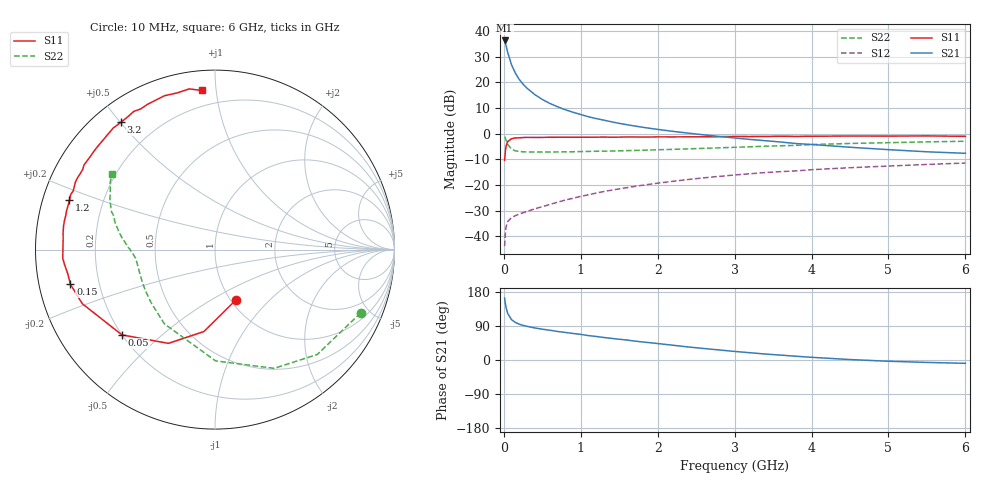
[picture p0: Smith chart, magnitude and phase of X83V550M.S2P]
! SIEMENS Small Signal Semiconductors
! BFP136W
! Si NPN RF Bipolar Junction Transistor in SOT343
! VCE = 3.5 V  IC = 50 mA
! Common Emitter S-Parameters:  September  1994
# GHz  S  MA  R  50
!  f  S11  S21  S12  S22
! GHz  MAG  ANG  MAG  ANG  MAG  ANG  MAG  ANG
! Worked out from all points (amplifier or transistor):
!   40 points, 10 MHz to 6 GHz, reference 50 ohm
!   highest |S21| = 36.4 dB at 10 MHz (marker M1)
!   |S21| within 3 dB of that: start of sweep to 36.94 MHz
!   unconditionally stable (mu >= 1): 683.3 MHz to 2.866 GHz
!   at 200 MHz: K = 0.54, MSG = 26.3 dB, |S12| = -31.3 dB
!   at 1.5 GHz: K = 1.11, MAG = 10.7 dB, |S12| = -21.5 dB
!   at 6 GHz: K = 0.96, MSG = 1.9 dB, |S12| = -11.4 dB
!   S11 on the Smith chart (normalised r, x): 10 MHz: 1.06, -0.65; 50 MHz: 0.20, -0.38; 150 MHz: 0.10, -0.12; 1.2 GHz: 0.08, +0.16; 3.2 GHz: 0.08, +0.50; 6 GHz: 0.11, +0.92
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0.01  0.3032 -67.2  66.02 163.4  0.0064 72.9  0.8846 -23.5
0.02  0.4607 -97.7  58.85 148.9  0.0115 62.2  0.8163 -45.7
0.03  0.5833 -116.4  51.7 137.7  0.0154 53.3  0.7392 -63.5
0.05  0.7033 -137.5  38.64 122.9  0.0193 40.0  0.62 -89.7
0.1  0.7983 -157.8  22.14 106.5  0.0231 32.6  0.5007 -124.3
0.15  0.8285 -166.5  15.21 99.1  0.0253 33.6  0.4627 -140.4
0.2  0.8319 -171.0  11.47 94.6  0.0271 33.8  0.4498 -149.5
0.25  0.8432 -174.5  9.261 91.4  0.0287 36.2  0.4442 -155.3
0.3  0.8494 -176.7  7.748 88.9  0.0303 38.5  0.4406 -159.3
0.4  0.8473 179.0  5.839 84.7  0.0343 42.4  0.4391 -164.4
0.5  0.8482 175.9  4.661 81.3  0.0377 45.7  0.4394 -167.7
0.6  0.8514 173.7  3.888 78.5  0.0418 48.3  0.4403 -169.8
0.7  0.8541 171.0  3.35 75.2  0.0462 51.2  0.4415 -171.3
0.9  0.8529 167.2  2.622 70.0  0.0551 53.6  0.4453 -173.9
1.1  0.8547 162.9  2.144 64.3  0.0645 55.6  0.4514 -175.4
1.2  0.8564 161.3  1.975 62.1  0.0695 56.2  0.4546 -176.2
1.7  0.8637 152.0  1.415 49.9  0.0937 56.2  0.4719 -179.8
2.2  0.8671 143.6  1.111 38.9  0.1182 53.9  0.4948 176.7
3.2  0.8819 126.5  0.774 19.2  0.1655 46.0  0.5558 167.7
4.5  0.9023 108.2  0.545 1.2  0.2173 34.2  0.6459 155.0
5.5  0.9068 99.1  0.444 -6.4  0.2513 26.4  0.6942 147.2
6  0.8893 94.6  0.415 -8.8  0.2682 22.0  0.7124 143.8
